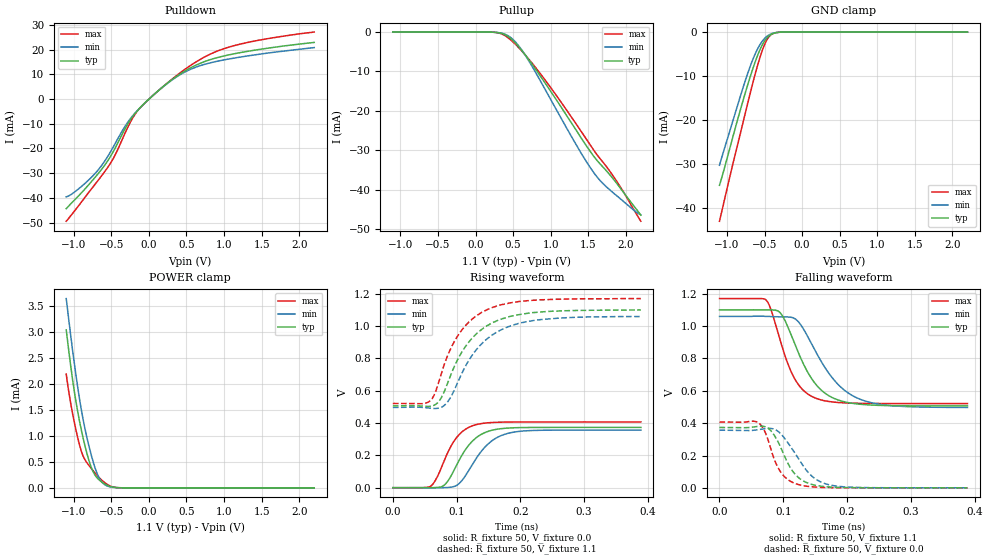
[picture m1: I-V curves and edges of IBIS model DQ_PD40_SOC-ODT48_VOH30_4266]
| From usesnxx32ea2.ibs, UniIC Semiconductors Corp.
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| DQ_PD40_SOC-ODT48_VOH30_4266
| (40 Ohm Pulldown, 48 Ohm System ODT Setting, VOH=VDDQ/3.0, 3200-4266Mbps)
[Model]   DQ_PD40_SOC-ODT48_VOH30_4266
Model_type   I/O
Vinl = 123.333mV
Vinh = 243.333mV
Vmeas = 183.333mV
Vref = 0.0mV
Cref = 0.0pF
Rref = 48.000Ohm
|   typ   min   max
|C_comp   0.834pF   0.784pF   0.884pF
C_comp_pullup   0.4170pF   0.3920pF   0.4420pF
C_comp_pulldown   0.4170pF   0.3920pF   0.4420pF
| Note: C_comp changes when the ODT circuit is enabled.
[Model Spec]
| Input threshold voltage corners
Vinl   0.1233V   0.1167V   0.1350V
Vinh   0.2433V   0.2367V   0.2550V
| Measurement voltage corners
Vmeas   0.1833V   0.1767V   0.1950V
| Timing spec test load voltage corners
Vref   0.0000V   0.0000V   0.0000V
| Dynamic Overshoot Parameters from LPDDR4 Specification
D_overshoot_ampl_h   0.30   NA   NA
D_overshoot_ampl_l   0.30   NA   NA
D_overshoot_area_h   0.1n   NA   NA
D_overshoot_area_l   0.1n   NA   NA
[Voltage Range]   1.1000V   1.0600V   1.1700V
[Pullup Reference]   1.1000V   1.0600V   1.1700V
| Junction Temperature (Ambient temp is 35C typ 95C min -40C max)
[Temperature Range]   50.0   110.0   -40.0
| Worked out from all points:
|   slope of the pulldown table from 0 to 0.165 V, typ, clamps not added: 37 ohm
|   slope of the pullup table from 0 to 0.165 V, typ, clamps not added: 15.6 kohm
|   GND clamp passes 1 mA (typ) near -0.45 V on its own axis
|   POWER clamp passes 1 mA (typ) near -0.88 V on its own axis
|   rising waveform, R_fixture 50, V_fixture 0.0: 20-80 % time 36ps typ, 40.3ps min, 31.8ps max; typ from 0 V to 0.373 V
|   falling waveform, R_fixture 50, V_fixture 1.1: 20-80 % time 45.6ps typ, 57.4ps min, 35.8ps max; typ from 1.1 V to 0.507 V
|   rising waveform, R_fixture 50, V_fixture 1.1: 20-80 % time 56.2ps typ, 59.5ps min, 51.8ps max; typ from 0.507 V to 1.1 V
|   falling waveform, R_fixture 50, V_fixture 0.0: 20-80 % time 30.9ps typ, 39.1ps min, 25.5ps max; typ from 0.373 V to 0.001 V
[Pulldown]
|   Voltage   I(typ)   I(min)   I(max)
-1.1V     -44.39mA   -39.58mA   -49.5mA
-888.8mV  -37.68mA   -35.17mA   -41.35mA
-664.4mV  -29.79mA   -28.29mA   -32.48mA
-479.6mV  -21.57mA   -19.68mA   -24.36mA
-291.5mV  -10.62mA   -9.821mA   -12.1mA
-152.9mV  -4.694mA   -4.619mA   -4.822mA
137.5mV   3.734mA    3.707mA    3.742mA
378.4mV   9.422mA    9.201mA    9.791mA
701.8mV   14.75mA    13.74mA    16.43mA
1.045V    17.81mA    16.16mA    20.89mA
1.471V    20.14mA    18.2mA     23.91mA
2.2V      22.98mA    20.89mA    27.18mA
[GND Clamp]
|   Voltage   I(typ)   I(min)   I(max)
-1.1V     -34.75mA   -30.21mA   -42.91mA
-944.9mV  -25.23mA   -21.44mA   -31.55mA
-803mV    -16.5mA    -13.5mA    -21.65mA
-727.1mV  -12.12mA   -9.513mA   -16.33mA
-671mV    -9.079mA   -6.866mA   -12.51mA
-598.4mV  -5.545mA   -4.01mA    -7.885mA
-525.8mV  -2.767mA   -1.975mA   -3.963mA
-473mV    -1.423mA   -1.031mA   -1.887mA
-416.9mV  -598.1uA   -441.3uA   -665.3uA
-357.5mV  -192.3uA   -144.5uA   -174.3uA
-251.9mV  -13.29uA   -11.93uA   -7.91uA
2.2V      0A         0A         0A
[Pullup]
|   Voltage   I(typ)   I(min)   I(max)
-1.1V     5.229uA    8.059uA    2.358uA
233.2mV   -40.51uA   -40.55uA   -42.22uA
335.5mV   -284.5uA   -237.4uA   -391.9uA
434.5mV   -1.159mA   -947.5uA   -1.465mA
550mV     -3.184mA   -2.927mA   -3.464mA
682mV     -6.308mA   -6.472mA   -6.26mA
1.045V    -16.32mA   -18.64mA   -15.27mA
1.391V    -26.44mA   -30.26mA   -24.79mA
1.566V    -31.33mA   -35.46mA   -29.76mA
1.685V    -34.02mA   -38.22mA   -32.77mA
1.887V    -38.56mA   -41.63mA   -38.07mA
2.2V      -46.44mA   -46.38mA   -47.99mA
[POWER Clamp]
|   Voltage   I(typ)   I(min)   I(max)
-1.1V     3.033mA    3.633mA    2.184mA
-1.041V   2.345mA    2.929mA    1.625mA
-977.9mV  1.723mA    2.241mA    1.161mA
-911.9mV  1.2mA      1.611mA    764.8uA
-852.5mV  818.1uA    1.148mA    543.8uA
-779.9mV  447.8uA    701.5uA    396.3uA
-710.6mV  232.2uA    359uA      273.1uA
-657.8mV  146.8uA    178.9uA    190.6uA
-595.1mV  80.76uA    68.29uA    109.2uA
-499.4mV  21.31uA    13.13uA    27.43uA
-397.1mV  2.394uA    1.592uA    2.118uA
2.2V      0A         0A         0A
[Ramp]
|   typ   min   max
| 20% - 80%
dV/dt_r   223.72m/36.03p   213.67m/40.33p   243.96m/31.77p
dV/dt_f   356.03m/45.63p   337.66m/57.36p   389.18m/35.80p
| 25% - 75%
|dV/dt_r   186.43m/28.69p   178.06m/32.18p   203.30m/25.20p
|dV/dt_f   296.69m/36.40p   281.38m/45.81p   324.32m/28.50p
R_load = 50
[Rising Waveform]
R_fixture = 50
V_fixture = 0.0
|   Time   V(typ)   V(min)   V(max)
0s        460.5uV    391.3uV    338.1uV
58ps      150.5uV    145.1uV    6.959mV
67ps      1.344mV    -450.1uV   48.07mV
79ps      11.62mV    295.9uV    152.8mV
91ps      71.21mV    3.437mV    256mV
104ps     170.6mV    26.43mV    328.9mV
130ps     307mV      177.2mV    389.7mV
155ps     355.3mV    289.4mV    403.6mV
189ps     371mV      343.8mV    406.6mV
389ps     373.3mV    356.5mV    406.9mV
[Falling Waveform]
R_fixture   = 50
V_fixture   = 1.1
V_fixture_min = 1.06
V_fixture_max = 1.17
|   Time   V(typ)   V(min)   V(max)
0s        1.1V       1.06V      1.17V
74ps      1.1V       1.06V      1.157V
96ps      1.079V     1.057V     901.9mV
114ps     929.7mV    1.053V     704.5mV
127ps     805.8mV    1.011V     622.3mV
148ps     655.8mV    863.7mV    559.3mV
182ps     549.4mV    656.3mV    529.1mV
221ps     516.7mV    547.2mV    522.6mV
272ps     508.2mV    507.4mV    521.5mV
389ps     506.6mV    497.2mV    521.4mV
[Rising Waveform]
R_fixture   = 50
V_fixture   = 1.1
V_fixture_min = 1.06
V_fixture_max = 1.17
|   Time   V(typ)   V(min)   V(max)
0s        506.5mV    496.8mV    521.3mV
58ps      503.6mV    492.2mV    536.2mV
67ps      515.5mV    490.3mV    594.5mV
80ps      588.9mV    507.3mV    755.6mV
95ps      737.8mV    593mV      894.4mV
112ps     863mV      737.9mV    994.2mV
130ps     948.1mV    849.3mV    1.061V
152ps     1.012V     934.1mV    1.109V
221ps     1.084V     1.035V     1.16V
389ps     1.1V       1.059V     1.17V
[Falling Waveform]
R_fixture = 50
V_fixture = 0.0
|   Time   V(typ)   V(min)   V(max)
0s        373.4mV    356.6mV    407mV
58ps      379.4mV    358.1mV    408.7mV
75ps      372.1mV    367.7mV    310.8mV
86ps      324.8mV    362.6mV    175.8mV
95ps      259.4mV    339mV      103.9mV
110ps     132.2mV    263.6mV    44.04mV
125ps     60.19mV    174.3mV    19.1mV
148ps     18.21mV    62.6mV     5.643mV
178ps     4.397mV    14.5mV     1.429mV
389ps     518.3uV    477.6uV    357.8uV
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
